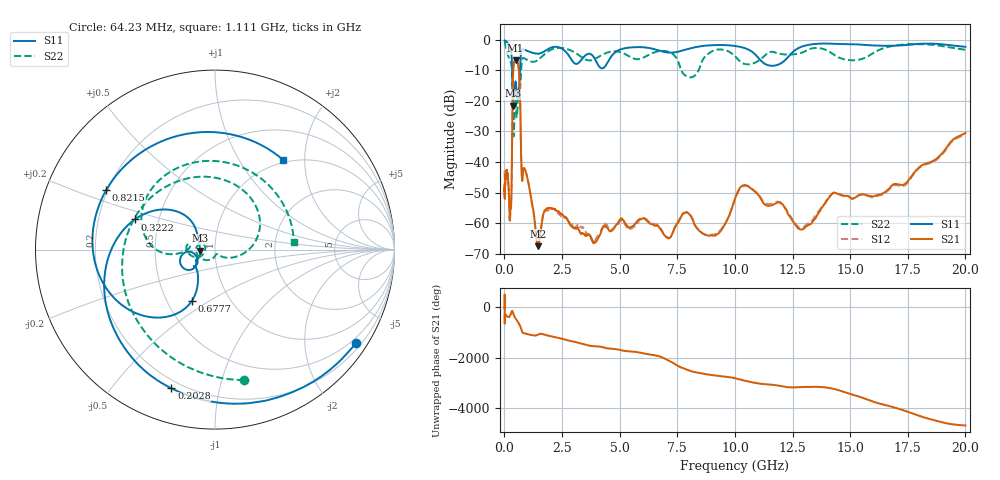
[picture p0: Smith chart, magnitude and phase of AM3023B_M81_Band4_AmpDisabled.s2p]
!Agilent Technologies,E8364B,MY43040894,A.07.50.67
!Agilent E8364B: A.07.50.67
!Date: Tuesday, October 27, 2020 10:38:55
!Correction: S11(Full 2 Port(1,2))
!S21(Full 2 Port(1,2))
!S12(Full 2 Port(1,2))
!S22(Full 2 Port(1,2))
!S2P File: Measurements: S11, S21, S12, S22:Log Frequency Sweep
# Hz S  dB  R 50
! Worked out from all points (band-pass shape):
!   3201 points, 10 MHz to 20 GHz, reference 50 ohm
!   highest |S21| = -6.83 dB at 482.5 MHz (marker M1); lowest = -67.4 dB at 1.446 GHz (marker M2)
!   |S21| within 3 dB of the highest: 386.2 MHz to 625.9 MHz (239.7 MHz wide, 47.4 % of centre)
!   lowest |S11| = -21.6 dB at 376 MHz (marker M3), VSWR 1.18, Z = 42.3 - j0.506 ohm
!   |S11| at or under -10 dB: 337.8 MHz to 677.8 MHz (340 MHz wide, 67 % of centre)
!   |S22| runs from -31.6 to -0.7 dB; largest |S21 - S12| = 0.011
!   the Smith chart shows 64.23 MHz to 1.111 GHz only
!   S11 on the Smith chart (normalised r, x): 64.23 MHz: 0.35, -3.26; 202.8 MHz: 0.16, -0.72; 322.2 MHz: 0.36, +0.16; 677.7 MHz: 0.66, -0.42; 821.5 MHz: 0.19, +0.25; 1.111 GHz: 0.96, +1.58
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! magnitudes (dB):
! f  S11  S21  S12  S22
! 10 MHz  -0.3  -49.1  -42.8  -0.8
! 35.55 MHz  -0.4  -47.0  -46.7  -1.4
! 64.23 MHz  -0.5  -43.5  -43.9  -2.6
! 126.1 MHz  -1.0  -43.5  -43.5  -4.6
! 202.8 MHz  -1.8  -52.6  -51.9  -6.1
! 247 MHz  -2.6  -57.5  -57.9  -6.8
! 322.2 MHz  -6.4  -43.1  -43.1  -9.1
! 376 MHz  -21.6  -11.5  -11.5  -25.8
! 447.2 MHz  -16.1  -7.0  -7.0  -22.1
! 482.5 MHz  -13.6  -6.8  -6.9  -19.6
! 677.7 MHz  -10.0  -18.0  -18.0  -16.5
! 750.6 MHz  -3.5  -43.8  -43.6  -7.5
! 821.5 MHz  -3.2  -42.2  -42.2  -6.0
! 1.111 GHz  -4.0  -49.5  -49.6  -7.1
! 1.446 GHz  -4.6  -67.4  -66.8  -6.7
! 1.59 GHz  -4.4  -61.7  -61.2  -5.8
! 5.639 GHz  -2.5  -60.4  -61.0  -6.3
! 8.053 GHz  -2.9  -57.3  -57.1  -12.3
! 9.068 GHz  -1.8  -63.9  -63.7  -3.6
! 10.51 GHz  -3.0  -47.6  -47.8  -8.1
! 13.01 GHz  -2.1  -61.5  -61.0  -3.9
! 20 GHz  -2.4  -30.4  -30.8  -3.4
